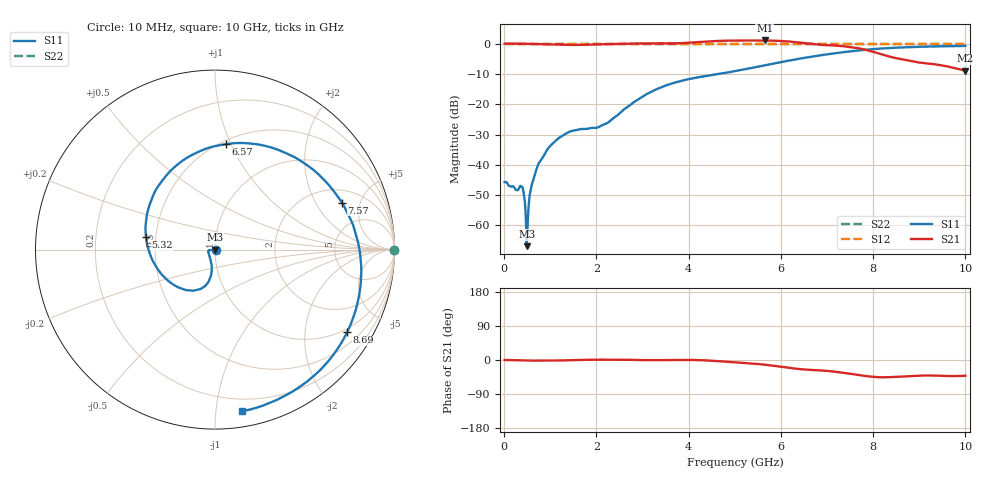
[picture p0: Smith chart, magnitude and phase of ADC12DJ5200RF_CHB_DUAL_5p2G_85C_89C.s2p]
! Texas Instruments, Inc.
! ADC12DJ5200RF - CH B S-Parameters (Dual Ch Mode, Fs = 5.2 GSPS, 85 degC case, 89 degC juntion)
! Port 1 represents the 100-ohm differenal input, Port 2 the digital output
! freq  dbS11  angS11  dbS21 angS21 dbS12 angS12 dbS22 angS22
# HZ S DB R 100
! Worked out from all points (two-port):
!   1000 points, 10 MHz to 10 GHz, reference 100 ohm
!   highest |S21| = 1.03 dB at 5.65 GHz (marker M1); lowest = -9.0 dB at 10 GHz (marker M2)
!   |S21| within 3 dB of the highest: start of sweep to 7.816 GHz
!   lowest |S11| = -66.8 dB at 490 MHz (marker M3), VSWR 1.00, Z = 100 + j0.0909 ohm
!   |S11| at or under -10 dB: start of sweep to 4.655 GHz
!   |S22| runs from 0.0 to 0.0 dB; largest |S21 - S12| = 0.77
!   S11 on the Smith chart (normalised r, x): 10 MHz: 1.01, -0.00; 5.32 GHz: 0.44, +0.07; 6.57 GHz: 0.53, +0.96; 7.57 GHz: 2.79, +3.39; 8.69 GHz: 0.87, -3.26; 10 GHz: 0.11, -1.18
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1e7  -45.69 -2.8  0.00 -0.0  0.00 0.0  0.00 0.0
3.8e8  -47.17 -16.4  -0.04 -1.1  0.00 0.0  0.00 0.0
4.9e8  -66.84 93.5  -0.08 -1.4  0.00 0.0  0.00 0.0
5.2e8  -56.15 -177.4  -0.09 -1.4  0.00 0.0  0.00 0.0
5.8e8  -47.93 -158.5  -0.11 -1.5  0.00 0.0  0.00 0.0
6.5e8  -44.16 -162.0  -0.16 -1.6  0.00 0.0  0.00 0.0
9.2e8  -35.36 -172.3  -0.25 -1.5  0.00 0.0  0.00 0.0
1.25e9  -30.53 -174.5  -0.39 -1.2  0.00 0.0  0.00 0.0
1.68e9  -28.19 -167.0  -0.42 0.2  0.00 0.0  0.00 0.0
2.22e9  -26.31 -127.8  -0.18 0.7  0.00 0.0  0.00 0.0
3.34e9  -14.84 -101.2  0.04 -0.4  0.00 0.0  0.00 0.0
4.23e9  -11.08 -126.9  0.51 -0.2  0.00 0.0  0.00 0.0
5.01e9  -9.07 -169.7  0.99 -6.3  0.00 0.0  0.00 0.0
5.32e9  -8.17 169.9  0.99 -8.8  0.00 0.0  0.00 0.0
5.65e9  -7.17 147.4  1.03 -12.4  0.00 0.0  0.00 0.0
6.57e9  -4.57 84.1  0.07 -25.4  0.00 0.0  0.00 0.0
6.67e9  -4.31 77.3  -0.11 -26.4  0.00 0.0  0.00 0.0
7.09e9  -3.36 49.3  -0.58 -29.7  0.00 0.0  0.00 0.0
7.57e9  -2.45 20.4  -1.26 -37.5  0.00 0.0  0.00 0.0
8.34e9  -1.48 -18.1  -4.24 -45.3  0.00 0.0  0.00 0.0
8.69e9  -1.23 -32.1  -5.41 -43.5  0.00 0.0  0.00 0.0
1e10  -0.78 -80.5  -8.98 -41.6  0.00 0.0  0.00 0.0
